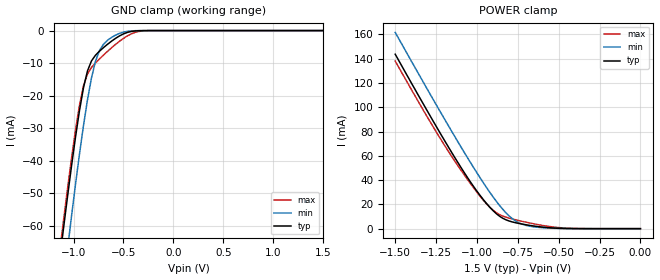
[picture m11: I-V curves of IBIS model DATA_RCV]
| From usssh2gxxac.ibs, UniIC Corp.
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|   Model DATA_RCV
[Model]  DATA_RCV
Model_type Input
Polarity   Non-Inverting
Vinl =   0.60000000V
Vinh =   0.90000000V
C_comp   1.6160pF   1.5990pF   1.6430pF
[Temperature Range]   25.0000   95.0000   0.0
[Voltage Range]   1.5000V   1.4000V   1.6000V
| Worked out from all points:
|   GND clamp passes 1 mA (typ) near -0.50 V on its own axis
|   POWER clamp passes 1 mA (typ) near -0.58 V on its own axis
[GND_clamp]
|Voltage   I(typ)   I(min)   I(max)
-1.5V     -169mA     -189.1mA   -163.8mA
-1.14V    -70.71mA   -88.3mA    -68.32mA
-1.1V     -60.74mA   -77.66mA   -58.33mA
-1.06V    -51.03mA   -67.22mA   -48.61mA
-1.02V    -41.65mA   -57.06mA   -39.27mA
-940mV    -24.55mA   -37.9mA    -22.88mA
-860mV    -12.39mA   -21.26mA   -13.32mA
-780mV    -7.577mA   -9.433mA   -9.942mA
-740mV    -6.329mA   -6.125mA   -8.71mA
-620mV    -3.273mA   -2.113mA   -5.305mA
-300mV    -11.81uA   -4.878uA   -91.71uA
1.5V      4.577nA    23.6nA     33.33nA
[POWER_clamp]
|Voltage   I(typ)   I(min)   I(max)
-1.5V     143.7mA    161.7mA    138.1mA
-1.22V    77.56mA    95.29mA    73.32mA
-1.12V    55.19mA    72.34mA    52.54mA
-1.02V    34.59mA    50.23mA    33.56mA
-960mV    23.77mA    37.63mA    23.28mA
-900mV    14.66mA    25.9mA     15mA
-840mV    8.415mA    15.63mA    10.28mA
-780mV    5.408mA    7.848mA    7.861mA
-700mV    3.206mA    2.693mA    5.332mA
-600mV    1.29mA     794.5uA    2.681mA
-420mV    69.47uA    44.47uA    238.7uA
0V        4.577nA    6.249nA    39.08nA
